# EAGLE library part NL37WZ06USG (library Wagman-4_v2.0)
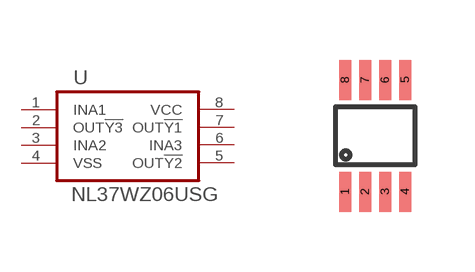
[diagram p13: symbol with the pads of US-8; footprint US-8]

Designator prefix U

## NL37WZ06USG  [US-8]
1  INA1  pwr
2  OUT!Y3  pas
3  INA2  pas
4  VSS  pas
5  OUT!Y2  pas
6  INA3  pas
7  OUT!Y1  pas
8  VCC  pas

## Footprint US-8 (pad centres in mm)
smd 0.3 x 1: 1 -0.75,-1.4; 2 -0.25,-1.4; 3 0.25,-1.4; 4 0.75,-1.4; 5 0.75,1.4; 6 0.25,1.4; 7 -0.25,1.4; 8 -0.75,1.4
